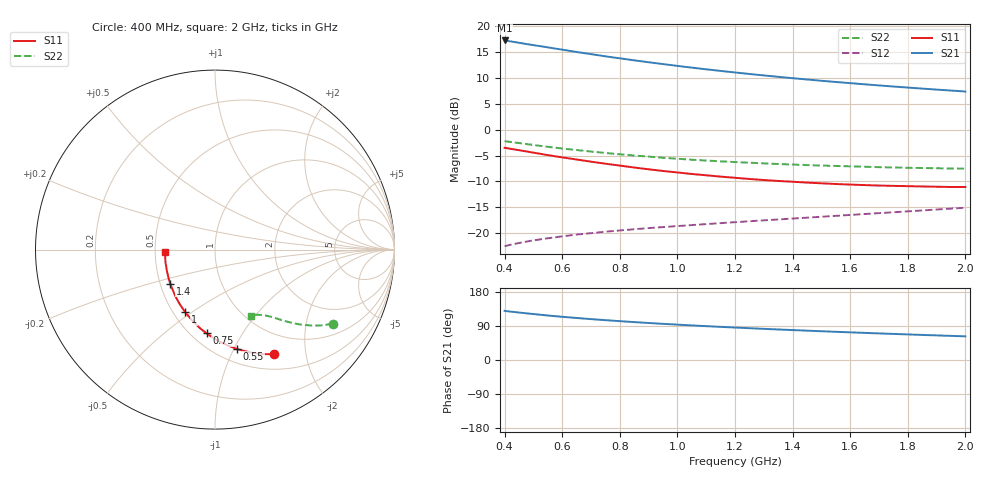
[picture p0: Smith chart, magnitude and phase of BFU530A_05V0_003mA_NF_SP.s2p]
! Filename:  P:\Prog\Test\Noise\ATS_data\Testdata_Net\06 Compressed Noise after Statistics\BFU530A_APG2013_33_A05_05p0V_003mA_NF_CM01_D.sf
! Date/Time: Tue 16/Apr/2013 15:10:56
! BFU530A_APG2013_33_A05_05p0V_1to25mA_NF_CM01_Bias3_R.sf
! Noise Parameter Data File
! BFU530A_APG2013_33_A05_05p0V_1to25mA_NF_CM01
! Date/time: Fri Apr 12 15:27:54 2013
! VAR V_out= 5.001000
! VAR I_out= 3.005000
! VAR V_in= 0.809400
! VAR I_in= 0.031510
! Device data file deembeded for feedlines and parallel
! Original file: \06 Compressed Noise after Statistics\BFU530A_APG2013_33_A05_05p0V_003mA_NF_CM01_R.sf
! Feed-files: PR017V01_150413_Feed1.s2p, PR017V01_150413_Feed2.s2p
! Parallel-file: PR017V01_150413_Par.s2p
# MHz S MA R 50
!  Freq-MHz  S11-mag  S11-arg  S21-mag  S21-arg  S12-mag  S12-arg  S22-mag  S22-arg
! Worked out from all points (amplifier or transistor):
!   37 points, 400 MHz to 2 GHz, reference 50 ohm
!   highest |S21| = 17.3 dB at 400 MHz (marker M1)
!   |S21| within 3 dB of that: start of sweep to 741.6 MHz
!   unconditionally stable (mu >= 1): 1.845 GHz to end of sweep
!   at 500 MHz: K = 0.44, MSG = 18.9 dB, |S12| = -21.4 dB
!   at 1.1 GHz: K = 0.80, MSG = 15.0 dB, |S12| = -18.3 dB
!   at 2 GHz: K = 1.01, MAG = 10.5 dB, |S12| = -15.1 dB
!   lowest NFmin = 0.52 dB at 440 MHz
!   S11 on the Smith chart (normalised r, x): 400 MHz: 0.70, -1.47; 550 MHz: 0.63, -1.03; 750 MHz: 0.59, -0.71; 1 GHz: 0.57, -0.47; 1.4 GHz: 0.56, -0.24; 2 GHz: 0.56, -0.02
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400  0.668 -60.6  7.305 129.7  0.07456 60.0  0.774 -32.2
420  0.6535 -63.0  7.158 127.8  0.07684 59.2  0.7608 -33.1
440  0.6396 -65.4  7.013 126.1  0.07899 58.4  0.7483 -34.0
480  0.6134 -69.8  6.713 122.8  0.08294 57.0  0.7234 -35.7
550  0.5675 -77.5  6.265 117.4  0.08886 55.1  0.6824 -38.3
600  0.5394 -82.4  5.948 114.0  0.09279 54.1  0.6575 -39.8
650  0.5144 -87.0  5.648 110.9  0.09652 53.3  0.6355 -41.1
700  0.4902 -91.5  5.386 107.9  0.09968 52.6  0.6141 -42.4
750  0.4686 -95.8  5.129 105.1  0.1029 52.1  0.595 -43.4
800  0.4491 -100.1  4.905 102.5  0.1059 51.8  0.578 -44.4
850  0.4303 -104.2  4.692 100.0  0.1087 51.5  0.562 -45.3
900  0.4136 -108.2  4.496 97.7  0.1116 51.3  0.5486 -46.1
950  0.3985 -111.9  4.314 95.4  0.1141 51.3  0.5348 -46.9
1000  0.3854 -115.6  4.145 93.3  0.1167 51.3  0.5233 -47.6
1100  0.3619 -122.8  3.84 89.3  0.1219 51.6  0.5024 -49.0
1200  0.3422 -129.8  3.58 85.7  0.1272 51.9  0.4858 -50.3
1300  0.3256 -136.3  3.352 82.2  0.1325 52.3  0.4721 -51.6
1400  0.3134 -142.8  3.151 79.0  0.1379 52.9  0.4597 -52.8
1500  0.3027 -149.1  2.974 75.9  0.1436 53.4  0.4495 -54.1
1650  0.2909 -157.9  2.749 71.6  0.1526 54.2  0.4378 -56.1
1750  0.2858 -163.7  2.617 68.8  0.1588 54.8  0.4308 -57.4
2000  0.2788 -176.8  2.342 62.4  0.1756 56.0  0.4192 -61.1
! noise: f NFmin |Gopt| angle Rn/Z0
400  0.5435  0.3977  22.14  0.1552
460  0.5188  0.3661  28.16  0.1494
600  0.644  0.3681  32.81  0.1579
800  0.6246  0.317  51.32  0.1272
1000  0.6731  0.2982  66.87  0.1168
1200  0.7292  0.2817  78.05  0.113
1400  0.7572  0.2627  95.43  0.1067
1600  0.8001  0.2707  111.9  0.0863
1800  0.7269  0.3277  134.2  0.0632
2000  0.7845  0.325  143.7  0.0608
